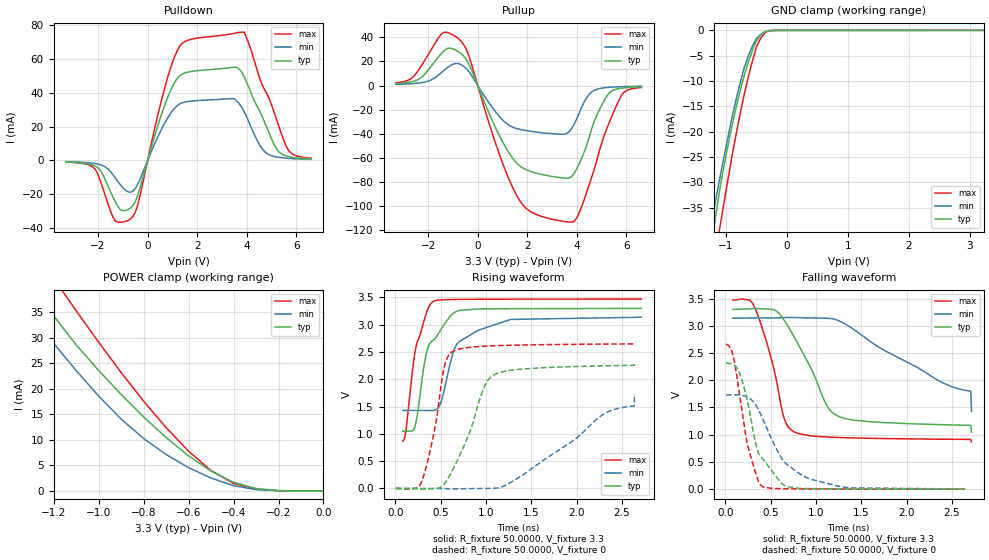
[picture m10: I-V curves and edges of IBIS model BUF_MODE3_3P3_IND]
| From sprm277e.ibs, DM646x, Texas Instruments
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|   Model Cell BUF_MODE3_3P3_IND
[Model]   BUF_MODE3_3P3_IND
Model_type   3-state
Polarity   Non-Inverting
Enable   Active-Low
Cref =  10.0000pF
Rref =  50.0000
Vref =  1.5V
Vmeas =  1.65
C_comp   2.460431p   2.393507p   2.515096p
[Temperature Range]   25   125   -40
[Voltage Range]   3.3   3.14   3.47
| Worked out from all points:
|   slope of the pulldown table from 0 to 0.495 V, typ, clamps not added: 20.3 ohm
|   slope of the pullup table from 0 to 0.495 V, typ, clamps not added: 20 ohm
|   GND clamp passes 1 mA (typ) near -0.43 V on its own axis
|   POWER clamp passes 1 mA (typ) near -0.34 V on its own axis
|   rising waveform, R_fixture 50.0000, V_fixture 3.3: 20-80 % time 225ps typ, 278ps min, 157ps max; typ from 1.05 V to 3.3 V
|   rising waveform, R_fixture 50.0000, V_fixture 0: 20-80 % time 309ps typ, 831ps min, 167ps max; typ from 0 V to 2.31 V
|   falling waveform, R_fixture 50.0000, V_fixture 3.3: 20-80 % time 393ps typ, 1.18ns min, 226ps max; typ from 3.3 V to 1.05 V
|   falling waveform, R_fixture 50.0000, V_fixture 0: 20-80 % time 247ps typ, 381ps min, 170ps max; typ from 2.31 V to 0 V
[POWER_clamp]
|   voltage   I(typ)   I(min)   I(max)
-3.3V     198.1mA    147.7mA    240.4mA
-1.367V   45.97mA    38.22mA    53.43mA
-1.267V   38.79mA    32.62mA    46.11mA
-1.167V   32.44mA    27.17mA    39.57mA
-1.133V   30.55mA    25.4mA     37.46mA
-1V       23.63mA    18.62mA    29.19mA
-800mV    14.53mA    10.29mA    17.61mA
-600mV    6.889mA    4.575mA    7.788mA
-500mV    3.882mA    2.519mA    3.994mA
-400mV    1.69mA     1.037mA    1.482mA
-300mV    474.6uA    246uA      358.7uA
0V        29.06nA    191nA      21.89nA
[Pulldown]
|   voltage   I(typ)   I(min)   I(max)
-3.3V     -857.2uA   -659.9uA   -881.3uA
-2.2V     -2.801mA   -1.657mA   -3.948mA
-1.3V     -24.62mA   -10.4mA    -35.76mA
-700mV    -28.2mA    -18.75mA   -34.64mA
-400mV    -20.75mA   -14.16mA   -26.43mA
600mV     28.95mA    19.58mA    37.89mA
1.3V      50.04mA    33.45mA    67.51mA
3.5V      55.11mA    36.5mA     75.1mA
3.9V      49.34mA    28.73mA    75.84mA
4.7V      23.23mA    5.494mA    42.26mA
5.6V      2.628mA    1.32mA     8.057mA
6.6V      939.2uA    661.2uA    1.322mA
[Pullup]
|   voltage   I(typ)   I(min)   I(max)
-3.3V     1.595mA    947.8uA    2.213mA
-2.6V     3.469mA    1.644mA    7.26mA
-1.4V     28.05mA    11.87mA    43.83mA
-800mV    28.34mA    18.31mA    39.25mA
-400mV    19.56mA    12.82mA    27.04mA
900mV     -42.68mA   -26.24mA   -58.65mA
1.7V      -66.76mA   -36.35mA   -95.59mA
3.8V      -75.32mA   -35.31mA   -113.4mA
4.5V      -42.51mA   -7.2mA     -82.15mA
5.2V      -8.944mA   -1.655mA   -36.06mA
5.9V      -1.922mA   -858.9uA   -5.592mA
6.6V      -1.015mA   -557.8uA   -1.66mA
[GND_clamp]
|   voltage   I(typ)   I(min)   I(max)
-3.3V     -226.9mA   -171.5mA   -272.4mA
-1.3V     -47.68mA   -41.9mA    -54.23mA
-1.233V   -41.93mA   -37.59mA   -48.9mA
-1.167V   -36.46mA   -33.33mA   -43.78mA
-1.1V     -31.26mA   -29.11mA   -38.87mA
-900mV    -18.81mA   -17.15mA   -24.75mA
-700mV    -8.866mA   -7.351mA   -12.63mA
-566.7mV  -3.999mA   -3.143mA   -6.07mA
-500mV    -2.027mA   -1.616mA   -3.279mA
-366.7mV  -316.4uA   -314.5uA   -560.6uA
-166.7mV  -7.25uA    -10.36uA   -7.758uA
3.233V    -25.89nA   4.216uA    -9.036nA
[Ramp]
| variable   typ   min   max
dV/dt_f  1.3624722/0.39653036n   1.035381/1.347331n   1.5751362/0.22722138n
dV/dt_r  1.3956058/0.31086435n  1.0437337/0.83248622n  1.6079984/0.16766824n
R_load = 50
[Rising Waveform]
R_fixture = 50.0000
V_fixture = 3.3
V_fixture_min = 3.14
V_fixture_max = 3.47
|   time   V(typ)   V(min)   V(max)
82.77ps   1.047V     1.428V     866.1mV
114.3ps   1.048V     1.43V      1.031V
230.5ps   1.236V     1.43V      2.613V
337.1ps   2.435V     1.429V     3.184V
415.2ps   2.711V     1.431V     3.422V
504.4ps   2.912V     1.584V     3.455V
669.3ps   3.239V     2.616V     3.463V
913.9ps   3.289V     2.899V     3.466V
1.275ns   3.294V     3.097V     3.468V
2.714ns   3.3V       3.14V      3.47V
[Rising Waveform]
R_fixture = 50.0000
V_fixture = 0
V_fixture_min = 0
V_fixture_max = 0
|   time   V(typ)   V(min)   V(max)
6.551ps   28.65uV    31.58uV    25.92uV
282.5ps   -11.28mV   63.7uV     93.29mV
419.8ps   -3.969mV   -536.3uV   966.4mV
539.5ps   82.05mV    -3.963mV   2.225V
632.4ps   337.2mV    -8.834mV   2.509V
978ps     1.848V     -788.5uV   2.605V
1.087ns   2.079V     3.758mV    2.614V
2.307ns   2.247V     1.371V     2.645V
2.636ns   2.256V     1.513V     2.648V
2.638ns   2.314V     1.731V     2.667V
[Falling Waveform]
R_fixture = 50.0000
V_fixture = 3.3
V_fixture_min = 3.14
V_fixture_max = 3.47
|   time   V(typ)   V(min)   V(max)
82.77ps   3.3V       3.14V      3.47V
320.7ps   3.318V     3.144V     3.345V
496.2ps   3.304V     3.144V     2.454V
646.5ps   3.106V     3.152V     1.309V
756.5ps   2.801V     3.152V     1.052V
1.108ns   1.569V     3.139V     959.5mV
1.23ns    1.351V     3.107V     950.4mV
2.349ns   1.186V     1.997V     918mV
2.707ns   1.172V     1.8V       913.6mV
2.714ns   1.047V     1.428V     866.1mV
[Falling Waveform]
R_fixture = 50.0000
V_fixture = 0
V_fixture_min = 0
V_fixture_max = 0
|   time   V(typ)   V(min)   V(max)
6.551ps   2.314V     1.731V     2.667V
79.94ps   2.294V     1.733V     2.479V
156.1ps   2.129V     1.73V      1.733V
252.4ps   1.538V     1.683V     759mV
347.1ps   747.7mV    1.51V      220.3mV
418.5ps   543.3mV    1.262V     39.51mV
634ps     89.07mV    534.3mV    8.696mV
934.4ps   9.644mV    185.5mV    4.124mV
1.381ns   5.193mV    23.51mV    1.871mV
2.638ns   28.65uV    31.58uV    25.92uV
